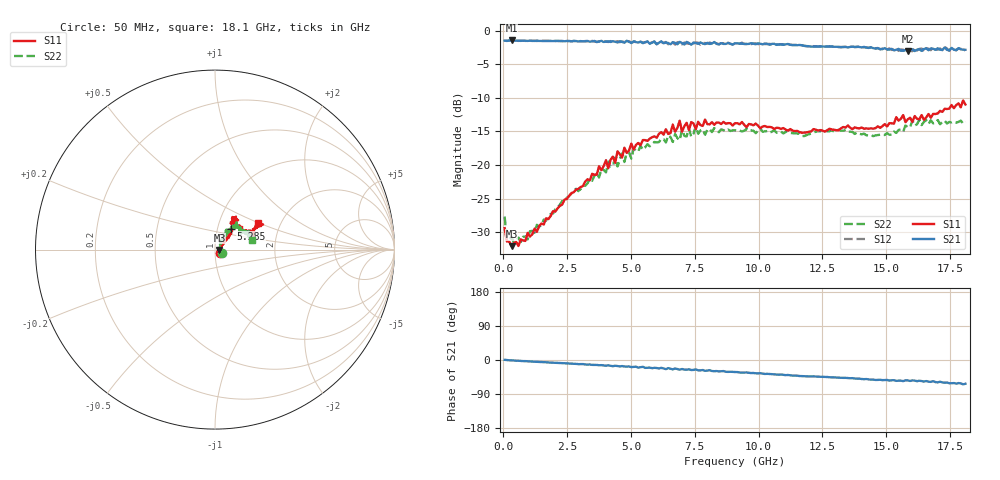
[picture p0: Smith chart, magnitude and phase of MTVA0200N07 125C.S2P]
! Network Analyzer HP8720D.06.14 Serial No. US36140669
! 21 Jun 2005  12:06:33
! Frequency  S11  S21  S12  S22
# HZ  S  DB R 50
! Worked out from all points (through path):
!   201 points, 50 MHz to 18.1 GHz, reference 50 ohm
!   highest |S21| = -1.45 dB at 320.8 MHz (marker M1); lowest = -3.0 dB at 15.84 GHz (marker M2)
!   group delay of S21, straight-line fit = 9.65 ps
!   lowest |S11| = -32.1 dB at 320.8 MHz (marker M3), VSWR 1.05, Z = 52.5 - j0.142 ohm
!   |S11| at or under -10 dB: start of sweep to end of sweep
!   |S22| runs from -31.5 to -13.3 dB; largest |S21 - S12| = 0.044
!   S11 on the Smith chart (normalised r, x): 50 MHz: 1.06, -0.04; 5.285 GHz: 1.16, +0.28; 18.1 GHz: 1.53, +0.50
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5e7  -29.41 -30.4  -1.46 0.5  -1.46 0.3  -27.69 -27.5
1.4025e8  -31.39 -17.8  -1.52 -0.2  -1.50 -0.4  -30.94 -13.4
3.2075e8  -32.10 -3.1  -1.45 -0.8  -1.47 -1.0  -30.77 -0.0
9.525e8  -30.12 14.1  -1.51 -3.5  -1.47 -3.6  -31.09 26.3
3.1185e9  -23.13 40.3  -1.57 -10.8  -1.60 -11.2  -23.05 56.7
4.021e9  -19.29 46.6  -1.63 -15.0  -1.60 -14.3  -21.10 55.6
4.11125e9  -20.50 46.9  -1.57 -14.1  -1.67 -15.3  -19.49 56.4
4.47225e9  -17.96 44.4  -1.76 -16.0  -1.55 -15.6  -20.22 61.3
4.65275e9  -18.88 44.9  -1.67 -16.1  -1.60 -17.5  -18.27 60.4
4.743e9  -17.42 48.7  -1.78 -17.2  -1.67 -16.5  -19.56 56.5
5.2845e9  -16.72 53.3  -1.75 -20.0  -1.77 -19.5  -18.02 51.9
6.09675e9  -15.34 53.1  -1.78 -22.3  -1.67 -22.2  -16.59 52.2
6.7285e9  -15.04 60.1  -1.81 -22.3  -2.06 -23.1  -15.40 47.2
6.909e9  -13.40 57.4  -1.65 -25.5  -1.68 -23.9  -16.31 48.2
6.99925e9  -15.04 56.6  -1.83 -23.8  -2.02 -25.9  -14.72 48.8
7.36025e9  -13.61 51.9  -2.07 -26.4  -1.73 -25.9  -15.80 52.1
7.54075e9  -14.65 54.7  -1.83 -24.8  -1.74 -27.9  -14.23 51.5
9.075e9  -13.76 59.4  -1.89 -31.7  -1.86 -32.1  -14.83 41.7
1.21435e10  -14.66 54.8  -2.35 -43.2  -2.29 -43.6  -15.18 43.4
1.512175e10  -13.78 29.2  -2.81 -54.2  -2.62 -54.1  -15.49 33.4
1.584375e10  -13.20 19.8  -3.04 -53.7  -2.82 -55.3  -14.36 34.8
1.81e10  -10.99 31.9  -2.83 -62.6  -2.98 -63.1  -13.52 14.0
